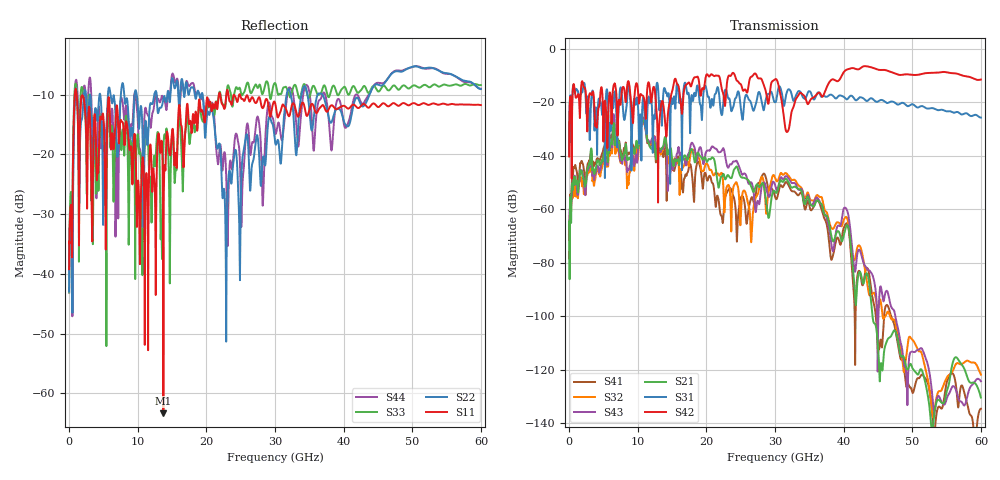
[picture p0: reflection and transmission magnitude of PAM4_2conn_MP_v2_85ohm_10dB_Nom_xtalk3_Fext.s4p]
! Info: Touchstone file created by Circ.  Input file=FAB50GbE_2conn_Midplane_Examax_Topo2_v2_85ohm_10dB_Nom.circ
# Hz S RI R 50
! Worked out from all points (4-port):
!   6000 points, 10 MHz to 60 GHz, reference 50 ohm
!   strongest paths, dB at 10 MHz, 15.01 GHz, 30.01 GHz, 45.01 GHz, 60 GHz:
!     S42: -40.2, -15.9, -11.3, -7.7, -11.4
!     S31: -39.8, -19.3, -19.9, -19.6, -25.6
!     S21: -64.6, -41.4, -53.4, -111.4, -130.5
!     S43: -78.5, -43.2, -51.0, -107.4, -124.4
!     S32: -69.2, -41.1, -48.1, -98.1, -121.9
!     S41: -68.5, -43.5, -55.2, -113.9, -134.7
!   lowest |S11| = -63.3 dB at 13.74 GHz (marker M1), VSWR 1.00, Z = 50.1 + j0.00221 ohm
!   |S11| at or under -10 dB: 1.113 GHz to 21.83 GHz (20.72 GHz wide, 181 % of centre); 23.21 GHz to 24.79 GHz (1.578 GHz wide, 6.57 % of centre); 24.89 GHz to end of sweep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
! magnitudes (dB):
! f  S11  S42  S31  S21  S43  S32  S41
! 10 MHz  -39.2  -40.2  -39.8  -64.6  -78.5  -69.2  -68.5
! 1.02 GHz  -9.2  -18.2  -15.0  -50.1  -50.6  -55.0  -44.9
! 13.74 GHz  -63.3  -20.9  -16.4  -36.2  -37.0  -37.2  -40.4
! 22.82 GHz  -11.0  -18.5  -15.1  -48.6  -41.1  -53.8  -54.8
! 31.68 GHz  -12.7  -31.0  -16.6  -48.7  -47.6  -46.6  -49.9
! 41.64 GHz  -11.8  -7.3  -18.9  -90.8  -83.3  -78.7  -103.4
! 60 GHz  -11.8  -11.4  -25.6  -130.5  -124.4  -121.9  -134.7
